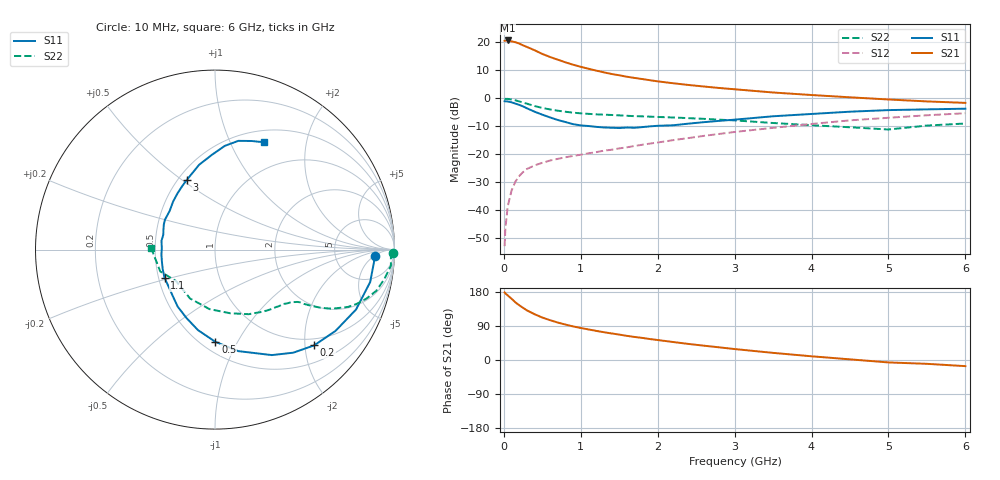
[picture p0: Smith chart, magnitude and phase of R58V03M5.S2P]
! SIEMENS Small Signal Semiconductors
! BFR183
! Si NPN RF Bipolar Junction Transistor in SOT23
! VCE = 8 V  IC = 3.5 mA
! Common Emitter S-Parameters:  May  1996
# GHz  S  MA  R  50
!  f  S11  S21  S12  S22
! GHz  MAG  ANG  MAG  ANG  MAG  ANG  MAG  ANG
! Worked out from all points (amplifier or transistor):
!   36 points, 10 MHz to 6 GHz, reference 50 ohm
!   highest |S21| = 20.7 dB at 50 MHz (marker M1)
!   |S21| within 3 dB of that: start of sweep to 357.6 MHz
!   unconditionally stable (mu >= 1): 1.225 GHz to 2.804 GHz
!   at 250 MHz: K = 0.32, MSG = 22.6 dB, |S12| = -26.3 dB
!   at 1.4 GHz: K = 1.05, MAG = 12.2 dB, |S12| = -18.3 dB
!   at 6 GHz: K = 0.87, MSG = 1.8 dB, |S12| = -5.3 dB
!   S11 on the Smith chart (normalised r, x): 10 MHz: 16, -5; 200 MHz: 0.85, -2.20; 500 MHz: 0.58, -0.82; 1.1 GHz: 0.54, -0.19; 3 GHz: 0.55, +0.52; 6 GHz: 0.64, +1.35
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0.01  0.8916 -2.3  10.72 178.2  0.0023 90.6  0.9917 -1.0
0.02  0.8882 -4.7  10.78 176.0  0.0047 86.5  0.9806 -2.0
0.05  0.8833 -11.8  10.87 170.5  0.0117 83.3  0.9841 -5.2
0.1  0.8539 -23.0  10.48 161.7  0.0226 78.1  0.9572 -10.0
0.15  0.81 -34.0  10.11 152.2  0.0327 72.2  0.9267 -14.4
0.2  0.7682 -44.0  9.566 144.5  0.0411 67.5  0.8858 -18.0
0.3  0.6675 -61.7  8.32 131.0  0.055 61.3  0.8072 -23.3
0.4  0.5803 -77.1  7.264 120.8  0.0638 56.2  0.7327 -26.7
0.5  0.5135 -89.8  6.244 112.0  0.0709 53.4  0.6764 -28.7
0.6  0.4587 -101.9  5.508 105.1  0.0779 51.8  0.6373 -29.8
0.7  0.413 -112.6  4.937 98.9  0.0834 51.4  0.6058 -30.7
0.8  0.3794 -123.3  4.424 93.5  0.0891 51.0  0.5797 -31.4
0.9  0.3476 -133.1  4.01 88.6  0.0941 51.8  0.5569 -31.8
1.1  0.3222 -150.7  3.394 80.7  0.1049 52.7  0.5311 -33.4
1.3  0.3035 -166.9  2.927 73.4  0.1167 53.4  0.5135 -34.9
1.6  0.3021 170.7  2.444 63.7  0.1343 54.9  0.4907 -38.0
2.2  0.3319 139.6  1.871 47.5  0.1799 55.8  0.4575 -46.3
3  0.4182 112.2  1.46 28.9  0.2518 52.0  0.4057 -62.5
3.5  0.4809 100.6  1.279 18.8  0.299 47.4  0.3646 -76.6
4.5  0.5806 84.6  1.049 1.7  0.4067 36.5  0.3058 -117.1
5.5  0.6388 71.3  0.886 -10.1  0.501 23.8  0.3283 -158.2
6  0.6568 65.6  0.834 -16.2  0.5454 15.4  0.357 178.2
